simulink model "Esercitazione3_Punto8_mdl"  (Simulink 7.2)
settings: Solver=ode45  StartTime=0.0  StopTime=10.0  RelTol=1e-3
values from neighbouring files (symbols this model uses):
  A = [-6.1   15.4    1.6    [Exercises08.m]
  B = [1; 0; 0]    [Exercises08.m]
  C = [0 10 10]    [Exercises08.m]
  Kyu = -inv(C*inv(A-B*K)*B)    [Exercises08.m]
  s1 = 5    [Exercises08.m]
  s2 = 20    [Exercises08.m]
  t1 = 0    [Exercises08.m]
  t2 = 10    [Exercises08.m]
  X0 = [7 -1 2]'    [Exercises08.m]
undefined symbols (not defined in the file or in its folder): K

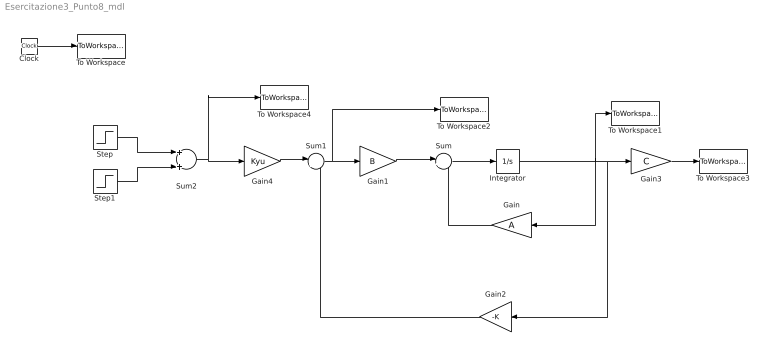
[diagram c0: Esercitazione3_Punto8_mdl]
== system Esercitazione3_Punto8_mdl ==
  Clock : Clock
  Gain : Gain  Orientation=left  Gain=A  Multiplication=Matrix(K*u)  ParameterDataType=sfix(16)  ParameterScaling=2^0  OutDataType=sfix(16)  OutScaling=2^0
  Gain1 : Gain  Gain=B  Multiplication=Matrix(K*u)  ParameterDataType=sfix(16)  ParameterScaling=2^0  OutDataType=sfix(16)  OutScaling=2^0
  Gain2 : Gain  Orientation=left  Gain=-K  Multiplication=Matrix(K*u)  ParameterDataType=sfix(16)  ParameterScaling=2^0  OutDataType=sfix(16)  OutScaling=2^0
  Gain3 : Gain  Gain=C  Multiplication=Matrix(K*u)  ParameterDataType=sfix(16)  ParameterScaling=2^0  OutDataType=sfix(16)  OutScaling=2^0
  Gain4 : Gain  Gain=Kyu  Multiplication=Matrix(K*u)  ParameterDataType=sfix(16)  ParameterScaling=2^0  OutDataType=sfix(16)  OutScaling=2^0
  Integrator : Integrator  InitialCondition=X0
  Step : Step  Time=t1  After=s1  SampleTime=0
  Step1 : Step  Time=t2  After=s2  SampleTime=0
  Sum : Sum  Inputs=|++  OutDataType=sfix(16)  OutScaling=2^0
  Sum1 : Sum  Inputs=|++  OutDataType=sfix(16)  OutScaling=2^0
  Sum2 : Sum  OutDataType=sfix(16)  OutScaling=2^0
  To Workspace : ToWorkspace  VariableName=time  SampleTime=-1  SaveFormat=Array
  To Workspace1 : ToWorkspace  VariableName=X  SampleTime=-1  SaveFormat=Array
  To Workspace2 : ToWorkspace  VariableName=u  SampleTime=-1  SaveFormat=Array
  To Workspace3 : ToWorkspace  VariableName=y  SampleTime=-1  SaveFormat=Array
  To Workspace4 : ToWorkspace  VariableName=yd  SampleTime=-1  SaveFormat=Array
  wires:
  Integrator/1 -> To Workspace1/1, Gain/1, Gain3/1, Gain2/1
  Sum/1 -> Integrator/1
  Clock/1 -> To Workspace/1
  Gain3/1 -> To Workspace3/1
  Gain1/1 -> Sum/1
  Gain/1 -> Sum/2
  Gain4/1 -> Sum1/1
  Sum1/1 -> Gain1/1, To Workspace2/1
  Gain2/1 -> Sum1/2
  Sum2/1 -> Gain4/1, To Workspace4/1
  Step/1 -> Sum2/1
  Step1/1 -> Sum2/2
